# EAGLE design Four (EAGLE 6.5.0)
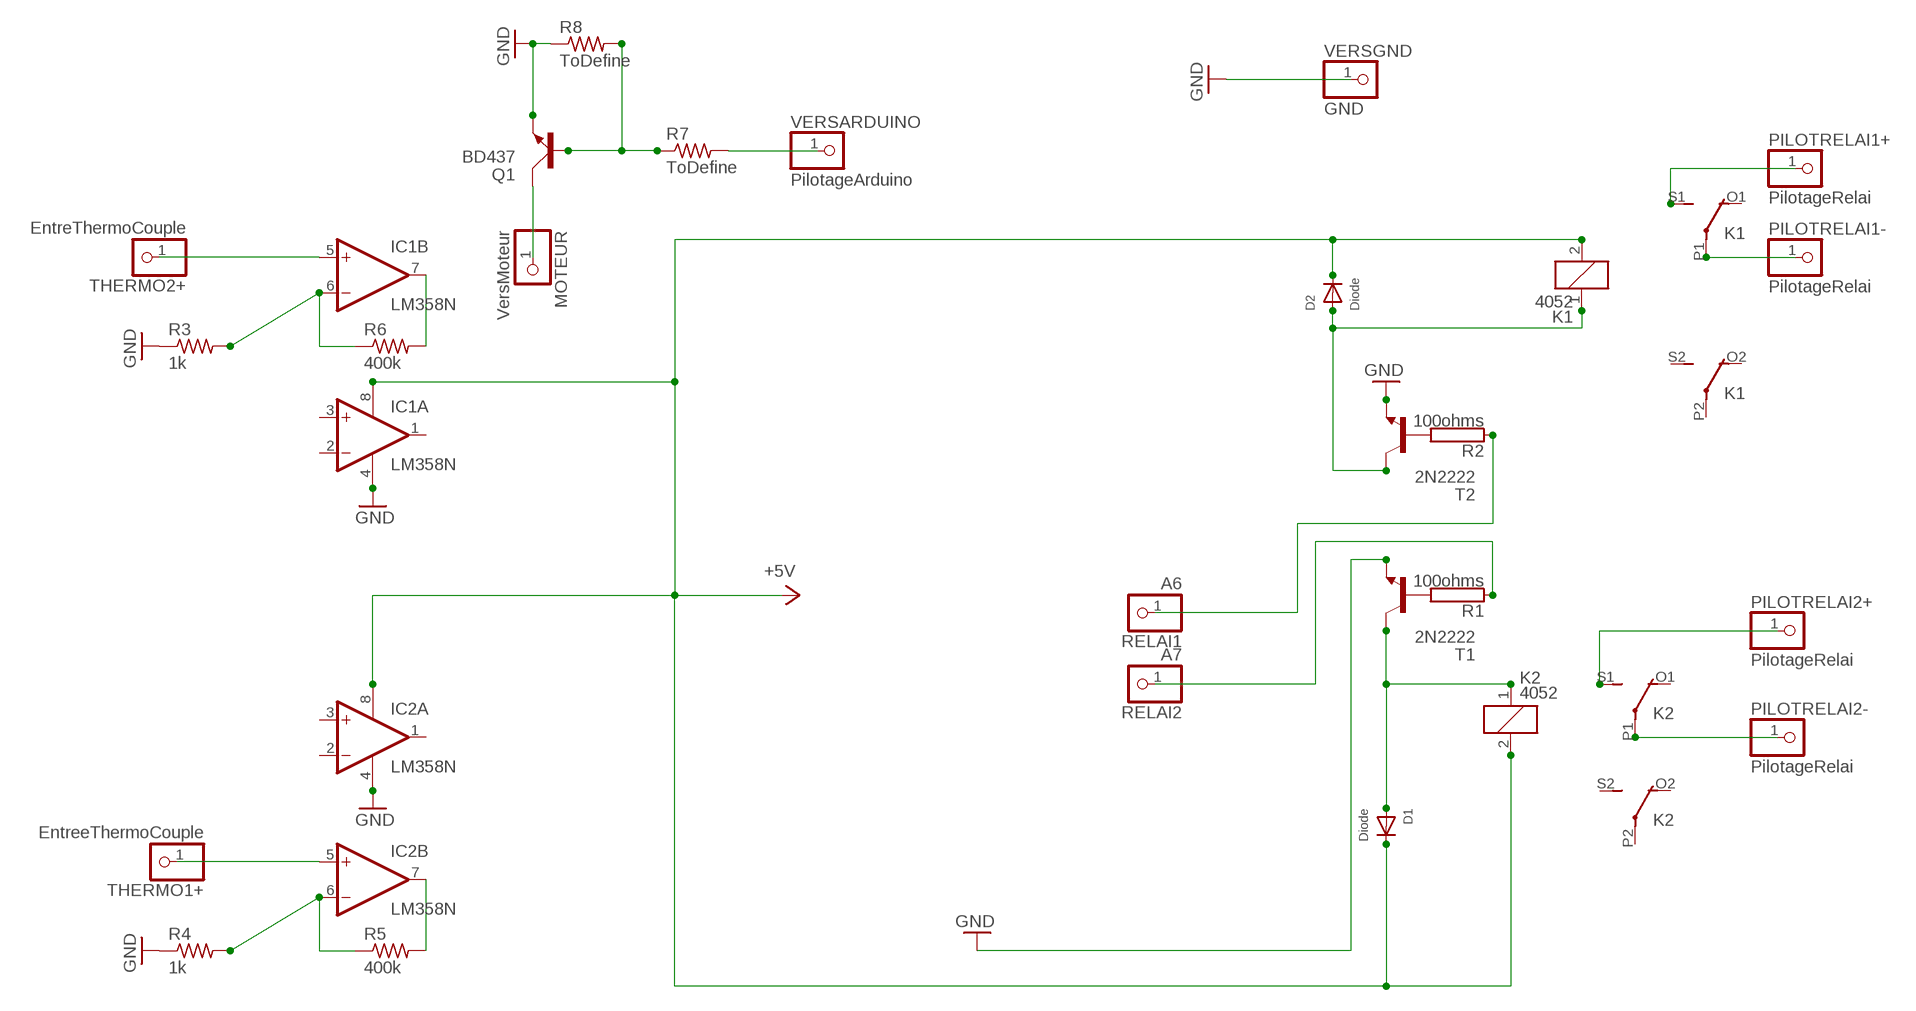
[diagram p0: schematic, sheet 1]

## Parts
D1  Diode  DIODEDO-1N4148  [DO-1N4148]
D2  Diode  DIODEDO-1N4148  [DO-1N4148]
IC1  LM358N  [DIL08]
IC2  LM358N  [DIL08]
K1  4052  [F4052]
K2  4052  [F4052]
MOTEUR  VersMoteur  PINHD-1X1  [1X01]
PILOTRELAI1+  PilotageRelai  PINHD-1X1  [1X01]
PILOTRELAI1-  PilotageRelai  PINHD-1X1  [1X01]
PILOTRELAI2+  PilotageRelai  PINHD-1X1  [1X01]
PILOTRELAI2-  PilotageRelai  PINHD-1X1  [1X01]
Q1  BD437  [TO126AV]
R1  100ohms  RAC01  [AC01]
R2  100ohms  RAC01  [AC01]
R3  1k  R-US_0411/12  [0411/12]
R4  1k  R-US_0411/12  [0411/12]
R5  400k  R-US_0411/12  [0411/12]
R6  400k  R-US_0411/12  [0411/12]
R7  ToDefine  R-US_0204/7  [0204/7]
R8  ToDefine  R-US_0204/7  [0204/7]
RELAI1  A6  PINHD-1X1  [1X01]
RELAI2  A7  PINHD-1X1  [1X01]
T1  2N2222  [TO92-EBC-OVAL]
T2  2N2222  [TO92-EBC-OVAL]
THERMO1+  EntreeThermoCouple  PINHD-1X1  [1X01]
THERMO2+  EntreThermoCouple  PINHD-1X1  [1X01]
VERSARDUINO  PilotageArduino  PINHD-1X1  [1X01]
VERSGND  GND  PINHD-1X1  [1X01]

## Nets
+5V: D1.C D2.C IC1.8(P:V+) IC2.8(P:V+) K1.2 K2.2
GND: IC1.4(P:V-) IC2.4(P:V-) Q1.E R3.1 R4.1 R8.1 T1.E T2.E VERSGND.1
N$1: R7.2 VERSARDUINO.1
N$2: D1.A K2.1 T1.C
N$3: IC1.6(B:-IN) R3.2 R6.1
N$4: R1.2 T1.B
N$5: R2.2 T2.B
N$6: R1.1 RELAI2.1
N$7: R2.1 RELAI1.1
N$8: IC2.6(B:-IN) R4.2 R5.1
N$9: D2.A K1.1 T2.C
N$10: IC1.5(B:+IN) THERMO2+.1
N$11: K1.S1(2:S) PILOTRELAI1+.1
N$12: K1.P1(2:P) PILOTRELAI1-.1
N$13: K2.S1(2:S) PILOTRELAI2+.1
N$14: IC2.5(B:+IN) THERMO1+.1
N$15: MOTEUR.1 Q1.C
N$16: Q1.B R7.1 R8.2
N$17: IC1.7(B:OUT) R6.2
N$18: IC2.7(B:OUT) R5.2
N$19: K2.P1(2:P) PILOTRELAI2-.1
Unconnected: IC1.1(A:OUT) IC1.2(A:-IN) IC1.3(A:+IN) IC2.1(A:OUT) IC2.2(A:-IN) IC2.3(A:+IN) K1.O1(2:O) K1.O2(3:O) K1.P2(3:P) K1.S2(3:S) K2.O1(2:O) K2.O2(3:O) K2.P2(3:P) K2.S2(3:S)

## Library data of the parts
D1 D2 = adafruit:DIODE: Diode
IC1 IC2 = linear:LM358: OP AMP also LM158; LM258; LM2904 Source: http://cache.national.com/ds/LM/LM158.pdf
K1 K2 = relay:4052: RELAY 2 x switch, Finder; OC_FARNELL: unknown; OC_NEWARK: unknown
MOTEUR PILOTRELAI1+ PILOTRELAI1- PILOTRELAI2+ PILOTRELAI2- RELAI1 RELAI2 THERMO1+ THERMO2+ VERSARDUINO VERSGND = pinhead:PINHD-1X1: PIN HEADER
Q1 = transistor-power:BD437: NPN TRANSISTOR
R1 R2 = resistor-power:R: Power Resitor; OC_FARNELL: unknown; OC_NEWARK: unknown
R3-R6 = resistor:R-US_: RESISTOR, American symbol
R7 R8 = adafruit:R-US_: RESISTOR, American symbol
T1 T2 = adafruit:2N2222: NPN TRANSISTOR Big oval pads

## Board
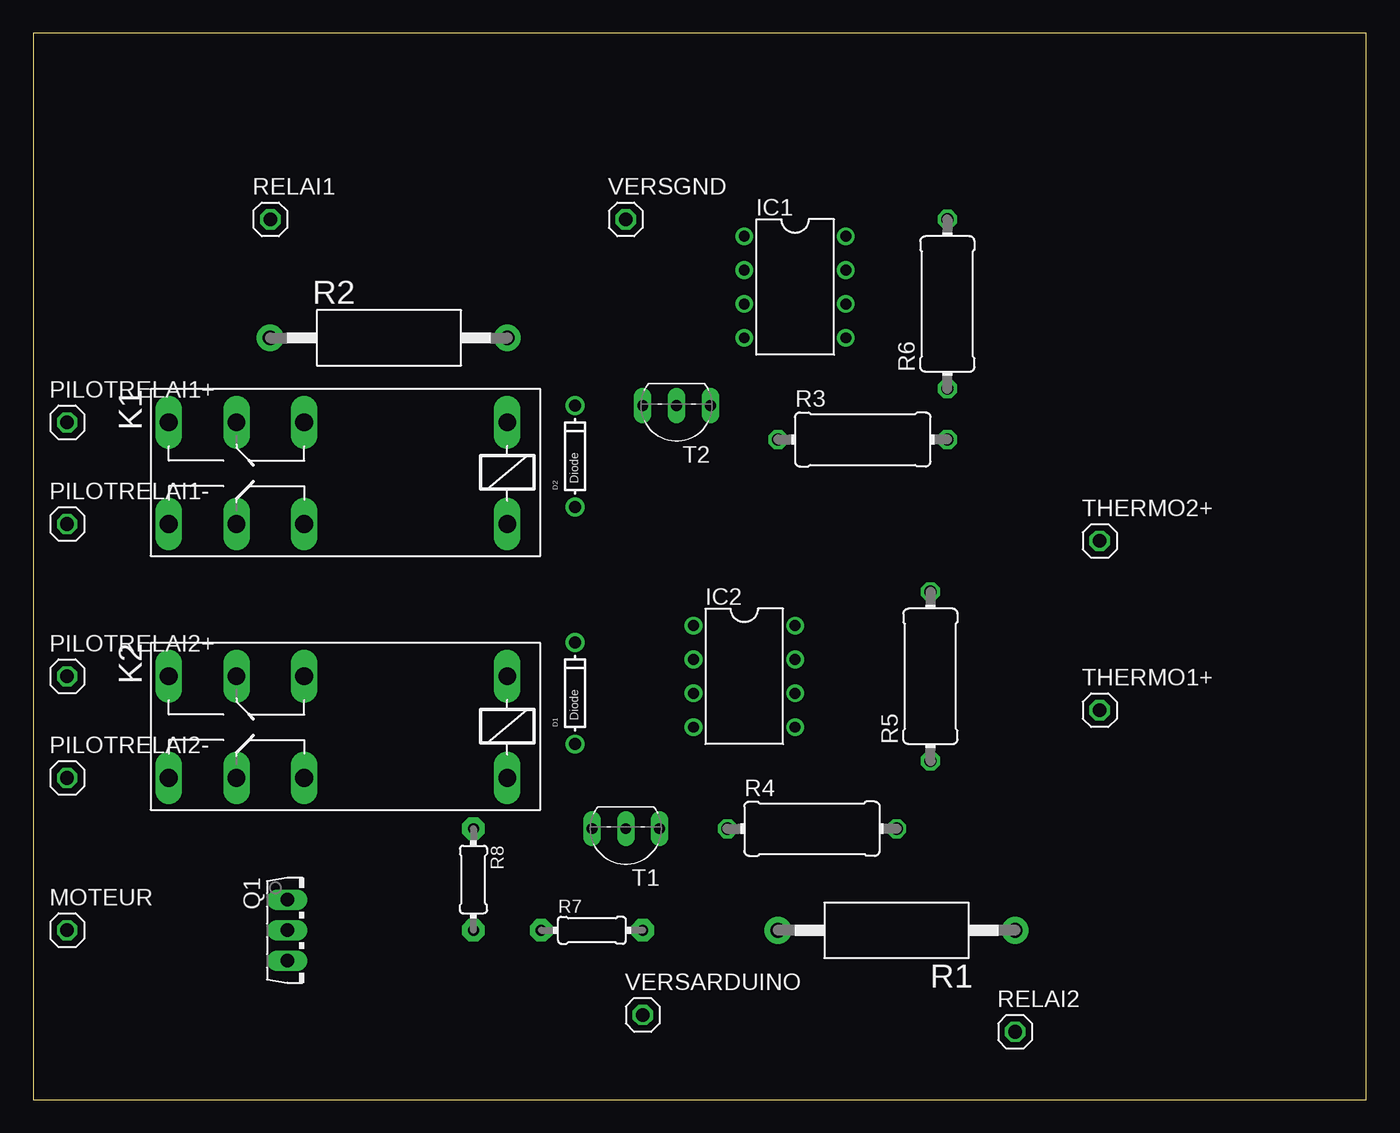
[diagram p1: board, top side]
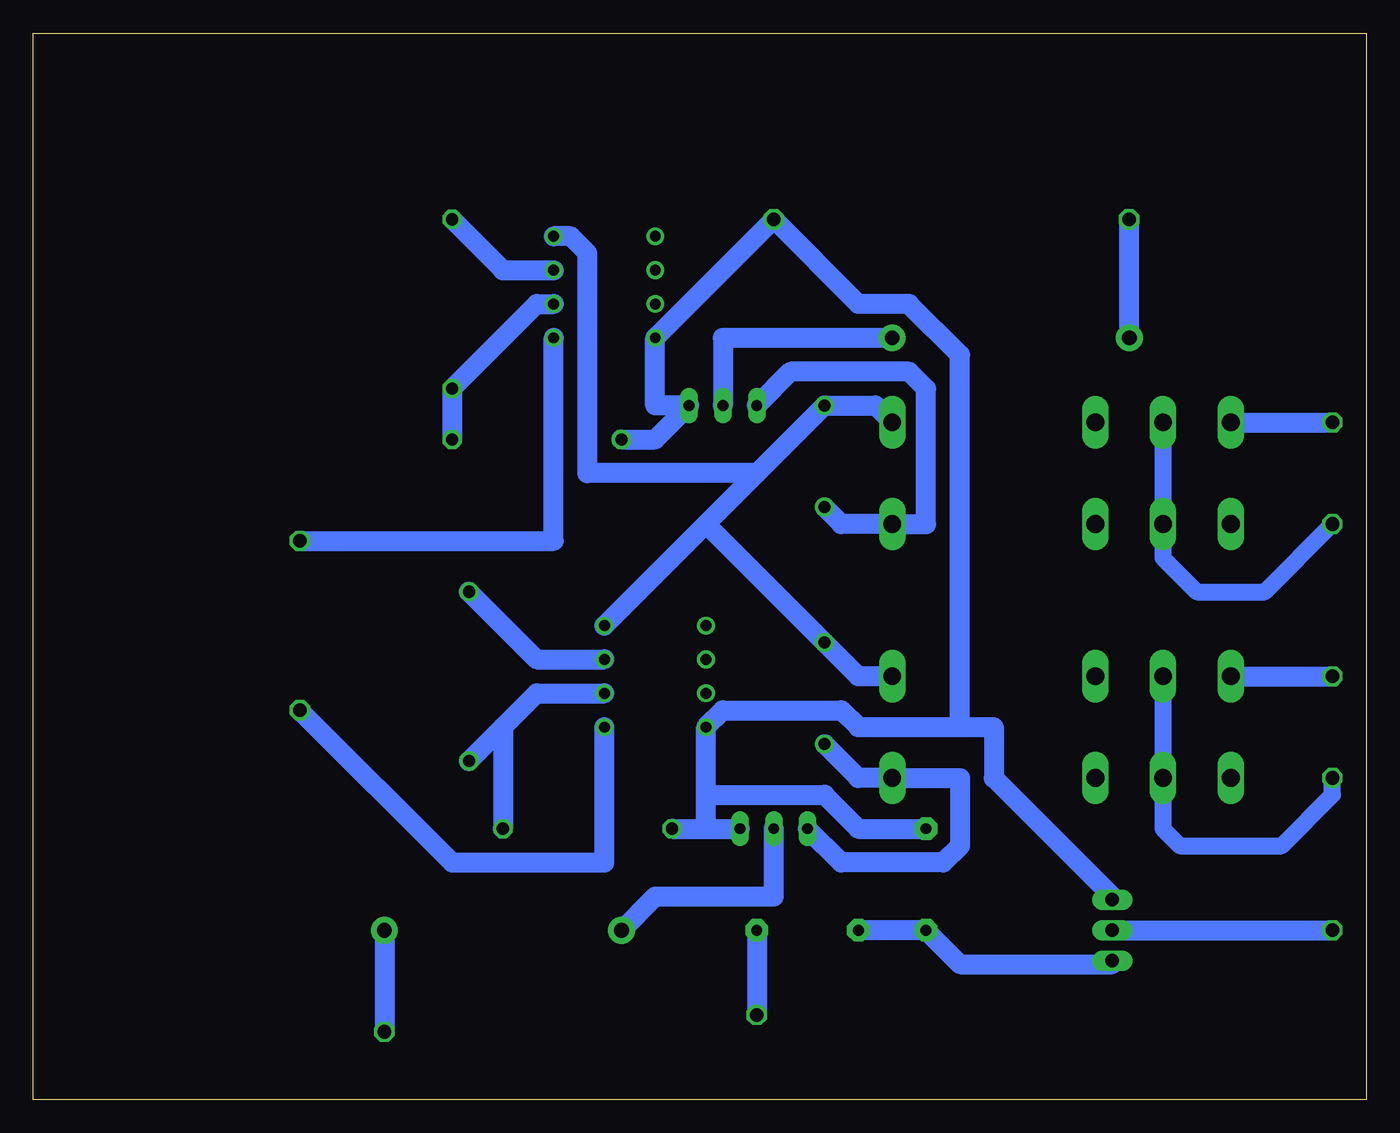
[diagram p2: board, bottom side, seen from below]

Size 100 x 80 mm. Coordinates in mm from the lower left corner, seen from the top.
Outline: 0,0 100,0 100,80 0,80 0,0
Copper layers (1*16): Top 0.035mm / dielectric 1.5mm / Bottom 0.035mm
Design rules "default *": minimum track width 1.5mm, minimum drill 24mil, track to track 12mil, track to pad 12mil, pad to pad 12mil, via to via 8mil, smd to smd 8mil, copper to edge 40mil, drill to drill 8mil, minimum pad ring 10mil, minimum via ring 8mil, stop-mask expansion 4mil, vias tented up to drill 0mil, thermal gap 10mil

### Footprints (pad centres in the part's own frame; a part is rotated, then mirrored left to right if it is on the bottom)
DO-1N4148 = drill 0.9: A -3.81,0; C 3.81,0
DIL08 = drill 0.813 pad 1.27: 1 -3.81,-3.81; 2 -1.27,-3.81; 3 1.27,-3.81; 4 3.81,-3.81; 5 3.81,3.81; 6 1.27,3.81; 7 -1.27,3.81; 8 -3.81,3.81
F4052 = drill 1.321 long: 1 -3.81,3.81; 2 -3.81,-3.81; O1 11.43,-3.81; O2 11.43,3.81; P1 16.51,-3.81; P2 16.51,3.81; S1 21.59,-3.81; S2 21.59,3.81
1X01 = drill 1.016 octagon: 1 0,0
TO126AV = drill 1.016 long: B 2.286,-1.27; C 0,-1.27; E -2.286,-1.27
AC01 = drill 1.1 pad 2: 1 -8.9,0; 2 8.9,0
0411/12 = drill 0.914 octagon: 1 -6.35,0; 2 6.35,0
0204/7 = drill 0.813 pad 1.676 octagon: 1 -3.81,0; 2 3.81,0
TO92-EBC-OVAL = drill 0.813 long: B 0,-1.27; C 2.54,-1.27; E -2.54,-1.27

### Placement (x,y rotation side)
D1  40.64,30.48 90 top
D2  40.64,48.26 90 top
IC1  57.15,60.96 270 top
IC2  53.34,31.75 270 top
K1  31.75,46.99 180 top
K2  31.75,27.94 180 top
MOTEUR  2.54,12.7 0 top
PILOTRELAI1+  2.54,50.8 0 top
PILOTRELAI1-  2.54,43.18 0 top
PILOTRELAI2+  2.54,31.75 0 top
PILOTRELAI2-  2.54,24.13 0 top
Q1  20.32,12.7 270 top
R1  64.77,12.7 180 top
R2  26.67,57.15 0 top
R3  62.23,49.53 0 top
R4  58.42,20.32 0 top
R5  67.31,31.75 90 top
R6  68.58,59.69 90 top
R7  41.91,12.7 0 top
R8  33.02,16.51 270 top
RELAI1  17.78,66.04 0 top
RELAI2  73.66,5.08 0 top
T1  44.45,19.05 180 top
T2  48.26,50.8 180 top
THERMO1+  80.01,29.21 0 top
THERMO2+  80.01,41.91 0 top
VERSARDUINO  45.72,6.35 0 top
VERSGND  44.45,66.04 0 top

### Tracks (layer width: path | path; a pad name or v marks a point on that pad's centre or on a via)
+5V
  Bottom 1.5: K2.2 38.1,31.75 D1.C 49.53,43.18 | 45.72,46.99 D2.C 36.83,52.07 K1.2 | 45.72,46.99 49.53,43.18 | 49.53,43.18 IC2.8 | IC1.8 59.69,64.77 58.42,63.5 58.42,46.99 45.72,46.99
GND
  Bottom 1.5: R3.1 53.34,49.53 T2.E 53.34,52.07 IC1.4 VERSGND.1 38.1,59.69 34.29,59.69 30.48,55.88 30.48,27.94 | R4.1 49.53,20.32 | 49.53,20.32 T1.E | 49.53,20.32 49.53,22.86 | 49.53,22.86 IC2.4 48.26,29.21 39.37,29.21 38.1,27.94 30.48,27.94 | 30.48,27.94 27.94,27.94 27.94,24.13 19.05,15.24 Q1.E | R8.1 38.1,20.32 40.64,22.86 49.53,22.86
N$1
  Bottom 1.5: R7.2 VERSARDUINO.1
N$2
  Bottom 1.5: T1.C 39.37,17.78 31.75,17.78 30.48,19.05 30.48,24.13 K2.1 38.1,24.13 D1.A
N$3
  Bottom 1.5: IC1.6 62.23,59.69 R6.1 R3.2
N$4
  Bottom 1.5: T1.B 44.45,15.24 53.34,15.24 R1.2
N$5
  Bottom 1.5: T2.B 48.26,57.15 R2.2
N$6
  Bottom 1.5: RELAI2.1 R1.1
N$7
  Bottom 1.5: RELAI1.1 R2.1
N$8
  Bottom 1.5: IC2.6 62.23,30.48 64.77,27.94 | R5.1 64.77,27.94 | 64.77,27.94 R4.2
N$9
  Bottom 1.5: T2.C 43.18,54.61 34.29,54.61 33.02,53.34 33.02,43.18 K1.1 39.37,43.18 D2.A
N$10
  Bottom 1.5: IC1.5 60.96,41.91 THERMO2+.1
N$11
  Bottom 1.5: K1.S1 PILOTRELAI1+.1
N$12
  Bottom 1.27: K1.P1 15.24,40.64 12.7,38.1 7.62,38.1 PILOTRELAI1-.1
N$13
  Bottom 1.5: K2.S1 PILOTRELAI2+.1
N$14
  Bottom 1.5: IC2.5 57.15,17.78 68.58,17.78 THERMO1+.1
N$15
  Bottom 1.5: Q1.C MOTEUR.1
N$16
  Bottom 1.5: Q1.B 19.05,10.16 30.48,10.16 R8.2 R7.1
N$17
  Bottom 1.5: IC1.7 64.77,62.23 R6.2
N$18
  Bottom 1.5: IC2.7 62.23,33.02 R5.2
N$19
  Bottom 1.27: K2.P1 15.24,20.32 13.97,19.05 6.35,19.05 2.54,22.86 PILOTRELAI2-.1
